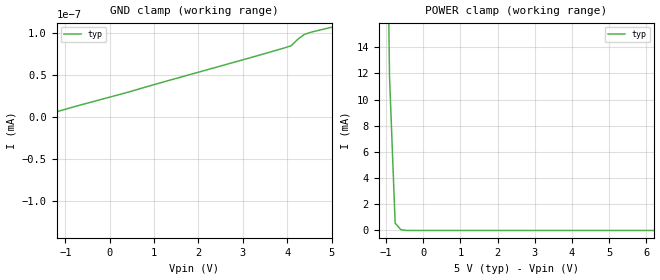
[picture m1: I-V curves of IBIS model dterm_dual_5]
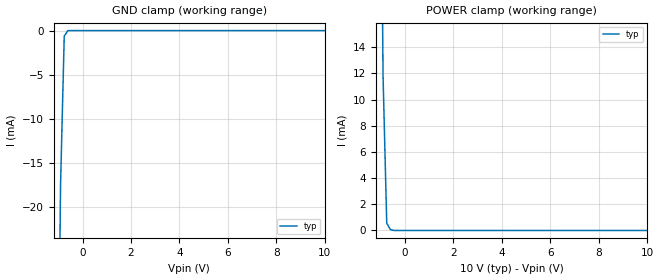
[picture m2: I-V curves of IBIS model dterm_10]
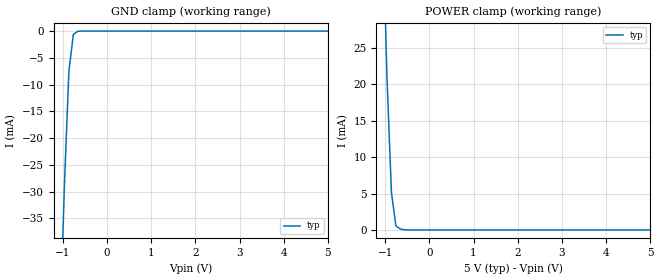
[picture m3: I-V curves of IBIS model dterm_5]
|Texas Instruments Incorporated
|tmux182, 1 Data Lane 8:1 24V Precision mux
[IBIS Ver]   4.1
[File name]   tmux182-sep.ibs
[Date]   06/29/26
[File Rev]   1.0
[Source]
| Texas Instruments Incorporated.
| ASC-INT-MUX
| 12500 TI Blvd
| Dallas, TX - 75243
[Notes]   Revision History:
| Rev 1.0: 06/29/2026
| - Initial version of the model
| - Model generated from simulations in SPECTRE
| - C_comp although listed in numerical order of value are
|   obtained from varying PVT conditions. For PVT conditions for
|   each specific value refer the buffer description under
|   respective [Model]. IBIS model user is responsible for using
|   appropriate C_comp to simulate for Signal Integrity.
[Disclaimer]
| This model is designed as an aid for customers of Texas Instruments.
| TI and its licensors and suppliers make no warranties, either expressed
| or implied, with respect to this  model, including the warranties of
| merchantability or fitness for a particular purpose. The model is
| provided solely on an "as is" basis. The entire risk as to its quality
| and performance is with the customer.
| This model is subject to change without notice. Texas Instruments
| Incorporated is not responsible for updating this model.
[Copyright]
(C) Copyright 2026 Texas Instruments Incorporated.All rights reserved.
|  Component TMUX182MDYY 16-pin - DYY package
|  Part # TMUX182MDYY
[Component]   TMUX182MDYY
[Manufacturer]  TI
[Package]
|   typ   min   max
R_pkg   0.0668   NA   NA
L_pkg   2.1992nH   NA   NA
C_pkg   0.2884pF   NA   NA
[Pin]   signal_name   model_name
   1   S4   sterm
   2   S6   sterm
   3   D   dterm
   4   S7   sterm
   5   S5   sterm
   6   ENZ   inbuf_n
   7   VEE   power
   8   GND   gnd
   9   A2   inbuf
   10   A1   inbuf
   11   A0   inbuf
   12   S3   sterm
   13   S0   sterm
   14   S1   sterm
   15   S2   sterm
   16   VDD   power
[Series Switch Groups]
On 1 /
On 2 /
On 3 /
On 4 /
On 5 /
On 6 /
On 7 /
On 8 /
Off 1 2 3 4 5 6 7 8 /
[Series Pin Mapping]  pin_2 model_name function_table_group
|  13   3   switch_dual_5   1
|  14   3   switch_dual_5   1
|  15   3   switch_dual_5   1
|  12   3   switch_dual_5   1
|   1   3   switch_dual_5   1
|   5   3   switch_dual_5   1
|   2   3   switch_dual_5   1
|   4   3   switch_dual_5   1
  13   3   switch_10   1
  14   3   switch_10   1
  15   3   switch_10   1
  12   3   switch_10   1
   1   3   switch_10   1
   5   3   switch_10   1
   2   3   switch_10   1
   4   3   switch_10   1
|  13   3   switch_5   1
|  14   3   switch_5   1
|  15   3   switch_5   1
|  12   3   switch_5   1
|   1   3   switch_5   1
|   5   3   switch_5   1
|   2   3   switch_5   1
|   4   3   switch_5   1
[Model Selector] dterm
dterm_dual_5 Use for operation at +/-5V
dterm_10 Use for operation at 10V
dterm_5 Use for operation at 5V
[Model Selector] sterm
sterm_dual_5 Use for operation at +/-5V
sterm_10 Use for operation at 10V
sterm_5 Use for operation at 5V
[Model Selector] inbuf_n
inbuf_n_dual_5 Use for operation at +/-5V
inbuf_n_10 Use for operation at 10V
inbuf_n_5 Use for operation at 5V
[Model Selector] inbuf
inbuf_dual_5 Use for operation at +/-5V
inbuf_10 Use for operation at 10V
inbuf_5 Use for operation at 5V
| switch_dual_5
[Model]   switch_dual_5
Model_type   Series_switch
|   typ   min   max
C_comp   4.014581e-12   NA   NA
[Voltage Range]   5   NA   NA
[Power Clamp Reference]   5   NA   NA
[Temperature Range]   27   NA   NA
[On]
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[Off]
|   typ   min   max
[R Series]   500G   NA   NA
| switch_10
[Model]   switch_10
Model_type   Series_switch
|   typ   min   max
C_comp   4.014581e-12   NA   NA
[Voltage Range]   10   NA   NA
[Power Clamp Reference]   10   NA   NA
[Temperature Range]   27   NA   NA
[On]
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[Off]
|   typ   min   max
[R Series]   500G   NA   NA
| switch_5
[Model]   switch_5
Model_type   Series_switch
|   typ   min   max
C_comp   4.014581e-12   NA   NA
[Voltage Range]   5   NA   NA
[Power Clamp Reference]   5   NA   NA
[Temperature Range]   27   NA   NA
[On]
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[Off]
|   typ   min   max
[R Series]   500G   NA   NA
| Models and submodels in the file (15): dterm_dual_5 (Terminator), dterm_10 (Terminator), dterm_5 (Terminator), switch_dual_5 (Series_switch), switch_10 (Series_switch), switch_5 (Series_switch), sterm_dual_5 (Terminator), sterm_10 (Terminator), sterm_5 (Terminator), inbuf_dual_5 (Input), inbuf_10 (Input), inbuf_5 (Input), inbuf_n_dual_5 (Input), inbuf_n_10 (Input), inbuf_n_5 (Input)
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| dterm_dual_5
[Model]   dterm_dual_5
Model_type   Terminator
|   typ   min   max
C_comp   6.362683e-12   NA   NA
[Voltage Range]   5   NA   NA
[Temperature Range]   27   NA   NA
[Power Clamp Reference]   5   NA   NA
[GND Clamp Reference]   0   NA   NA
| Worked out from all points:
|   GND clamp passes 1 mA (typ) near -5.76 V on its own axis
|   POWER clamp passes 1 mA (typ) near -0.76 V on its own axis
[GND Clamp]
|   Voltage   I(typ)   I(min)   I(max)
-10V      -3.643A    NA         NA
-5.455V   -30.47nA   NA         NA
-5.303V   -84.49pA   NA         NA
-5.152V   -60.21pA   NA         NA
-4.394V   -48.53pA   NA         NA
-3.939V   -34.13pA   NA         NA
-1.818V   -2.792pA   NA         NA
-1.667V   -5.674pA   NA         NA
-1.515V   1.66pA     NA         NA
3.939V    82.28pA    NA         NA
4.394V    98.48pA    NA         NA
5V        106.8pA    NA         NA
[POWER Clamp]
|   Voltage   I(typ)   I(min)   I(max)
-5V       2.031A     NA         NA
-1.061V   43.91mA    NA         NA
-909.1mV  11.75mA    NA         NA
-757.6mV  561.7uA    NA         NA
-606.1mV  63.16uA    NA         NA
-303mV    751pA      NA         NA
10V       -58.07pA   NA         NA
| dterm_10
[Model]   dterm_10
Model_type   Terminator
|   typ   min   max
C_comp   6.362683e-12   NA   NA
[Voltage Range]   10   NA   NA
[Temperature Range]   27   NA   NA
[Power Clamp Reference]   10   NA   NA
[GND Clamp Reference]   0   NA   NA
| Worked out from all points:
|   GND clamp passes 1 mA (typ) near -0.76 V on its own axis
|   POWER clamp passes 1 mA (typ) near -0.76 V on its own axis
[GND Clamp]
|   Voltage   I(typ)   I(min)   I(max)
-5V       -3.643A    NA         NA
-1.061V   -55.46mA   NA         NA
-909.1mV  -17.41mA   NA         NA
-757.6mV  -623.4uA   NA         NA
-606.1mV  -5.763uA   NA         NA
10V       106.8pA    NA         NA
[POWER Clamp]
|   Voltage   I(typ)   I(min)   I(max)
-5V       2.031A     NA         NA
-1.061V   43.91mA    NA         NA
-909.1mV  11.75mA    NA         NA
-757.6mV  561.7uA    NA         NA
-606.1mV  63.17uA    NA         NA
-303mV    751pA      NA         NA
10V       -58.07pA   NA         NA
| dterm_5
[Model]   dterm_5
Model_type   Terminator
|   typ   min   max
C_comp   6.362683e-12   NA   NA
[Voltage Range]   5   NA   NA
[Temperature Range]   27   NA   NA
[Power Clamp Reference]   5   NA   NA
[GND Clamp Reference]   0   NA   NA
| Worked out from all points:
|   GND clamp passes 1 mA (typ) near -0.76 V on its own axis
|   POWER clamp passes 1 mA (typ) near -0.77 V on its own axis
[GND Clamp]
|   Voltage   I(typ)   I(min)   I(max)
-5V       -3.643A    NA         NA
-1.061V   -55.46mA   NA         NA
-959.6mV  -28.6mA    NA         NA
-858.6mV  -7.403mA   NA         NA
-757.6mV  -623.4uA   NA         NA
-656.6mV  -32.47uA   NA         NA
5V        53.43pA    NA         NA
[POWER Clamp]
|   Voltage   I(typ)   I(min)   I(max)
-5V       2.031A     NA         NA
-1.061V   43.91mA    NA         NA
-959.6mV  21mA       NA         NA
-858.6mV  5.169mA    NA         NA
-757.6mV  561.5uA    NA         NA
-656.6mV  120.2uA    NA         NA
-454.6mV  1.693uA    NA         NA
5V        -29.79pA   NA         NA
